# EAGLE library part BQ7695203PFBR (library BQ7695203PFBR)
Battery Management 3-s to 16-s high-accuracy battery monitor and protector for Li-ion, Li-polymer and LiFePO4 Source: Datasheet
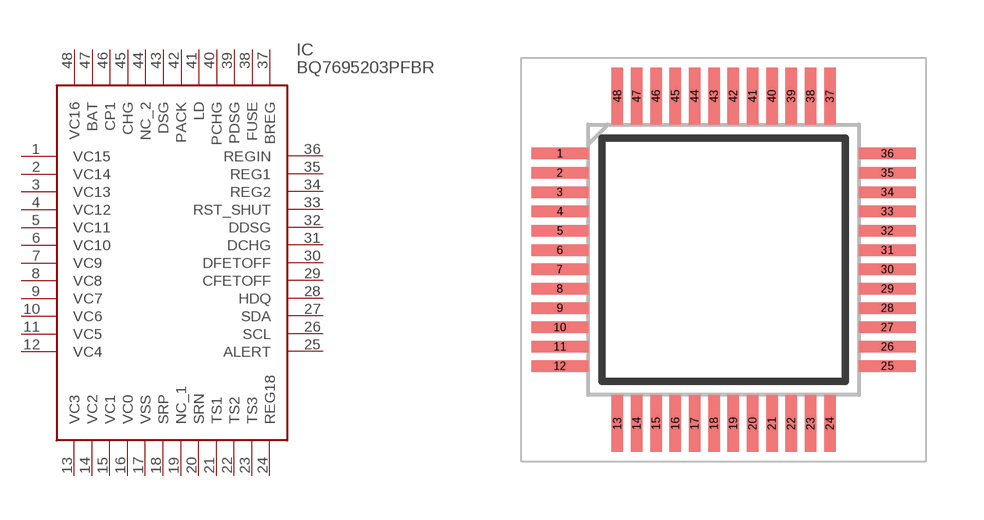
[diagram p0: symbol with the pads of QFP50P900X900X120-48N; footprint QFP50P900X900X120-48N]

Designator prefix IC

## BQ7695203PFBR (Description: Battery Management 3-s to 16-s high-accuracy battery monitor and protector for Li-ion, Li-polymer and LiFePO4; Height: 1.2mm; Manufacturer_Name: Texas Instruments; Manufacturer_Part_Number: BQ7695203PFBR; Mouser_Part_Number: 595-BQ7695203PFBR; Mouser_Price-Stock: https://www.mouser.co.uk/ProductDetail/Texas-Instruments/BQ7695203PFBR?qs=iLbezkQI%252Bsg2rrpTwJo3bg%3D%3D)  [QFP50P900X900X120-48N]
1  VC15
2  VC14
3  VC13
4  VC12
5  VC11
6  VC10
7  VC9
8  VC8
9  VC7
10  VC6
11  VC5
12  VC4
13  VC3
14  VC2
15  VC1
16  VC0
17  VSS
18  SRP
19  NC_1
20  SRN
21  TS1
22  TS2
23  TS3
24  REG18
25  ALERT
26  SCL
27  SDA
28  HDQ
29  CFETOFF
30  DFETOFF
31  DCHG
32  DDSG
33  RST_SHUT
34  REG2
35  REG1
36  REGIN
37  BREG
38  FUSE
39  PDSG
40  PCHG
41  LD
42  PACK
43  DSG
44  NC_2
45  CHG
46  CP1
47  BAT
48  VC16

## Footprint QFP50P900X900X120-48N (pad centres in mm)
PFB (S-PQFP-G48) HEIGHT 1.2
smd 1.475 x 0.3: 1 -4.238,2.75; 2 -4.238,2.25; 3 -4.238,1.75; 4 -4.238,1.25; 5 -4.238,0.75; 6 -4.238,0.25; 7 -4.238,-0.25; 8 -4.238,-0.75; 9 -4.238,-1.25; 10 -4.238,-1.75; 11 -4.238,-2.25; 12 -4.238,-2.75; 25 4.238,-2.75; 26 4.238,-2.25; 27 4.238,-1.75; 28 4.238,-1.25; 29 4.238,-0.75; 30 4.238,-0.25; 31 4.238,0.25; 32 4.238,0.75; 33 4.238,1.25; 34 4.238,1.75; 35 4.238,2.25; 36 4.238,2.75
smd 0.3 x 1.475: 13 -2.75,-4.238; 14 -2.25,-4.238; 15 -1.75,-4.238; 16 -1.25,-4.238; 17 -0.75,-4.238; 18 -0.25,-4.238; 19 0.25,-4.238; 20 0.75,-4.238; 21 1.25,-4.238; 22 1.75,-4.238; 23 2.25,-4.238; 24 2.75,-4.238; 37 2.75,4.238; 38 2.25,4.238; 39 1.75,4.238; 40 1.25,4.238; 41 0.75,4.238; 42 0.25,4.238; 43 -0.25,4.238; 44 -0.75,4.238; 45 -1.25,4.238; 46 -1.75,4.238; 47 -2.25,4.238; 48 -2.75,4.238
